|   Analog Devices INC.
|   IBIS Model of BF527/BF525/BF523
|   Embedded processor
|   208 Pin 17x17 CSP_BGA
[IBIS ver]   3.2
[File name]   bf527_1p8_17x17.ibs
[File Rev]   1.0
[Date]   02/23/2009
[Source]   From running Hspice on 90nm spice models.
[Notes]
|   Model data reflects 1.8v I/O Operation
|   No models exist for the following pins (Using type NC as
|   a placeholder):
|   XTAL, CLKIN, RTXI, RTXO, USB_ID, USB_DP, USB_XTALOUT,
|   USB_VBUS, USB_DM, VRSEL, USB_XTALIN, VROUT/EXT_WAKE1,
|   SS/PG, USB_RSET, USB_VREF
[Disclaimer]
|   This IBIS model is provided "AS IS, WHERE IS", AND WITH NO WARRANTY OF
|   ANY KIND EITHER EXPRESSED OR IMPLIED, INCLUDING BUT NOT LIMITED TO ANY
|   IMPLIED WARRANTIES OF MERCHANTABILITY AND FITNESS FOR A PARTICULAR
|   PURPOSE.  IN NO EVENT WILL ADI BE LIABLE FOR SPECIAL, COLLATERAL,
|   INCIDENTAL, OR CONSEQUENTIAL DAMAGES IN CONNECTION WITH OR ARISING OUT
|   OF THE USE OF THIS IBIS MODEL, AND IN NO EVENT SHALL ADI'S TOTAL
|   LIABILITY EXCEED $1,000, REGARDLESS OF THE BASIS FOR CLAIM.  ADI
|   RESERVES THE right to make changes to the products and IBIS models
|   without prior notice.
[Copyright]   This model is exclusive property of Analog Devices Inc
|   and is not to be resold or redistributed without the written
|   permission of Analog Devices.
|   Copyright (C)2008 Analog Devices, All Rights Reserved
[Component]   BF527/BF525/BF523
[Manufacturer] ANALOG DEVICES
[Package]
| variable   typ   min   max
R_pkg   217.00m   NA   NA
L_pkg   6.17nH   NA   NA
C_pkg   1.08pF   NA   NA
[Pin]   signal_name   model_name   R_pin   L_pin   C_pin
A1   GND   GND   NA   NA   NA
A2   PF9   prw0812swcdg_25   NA   NA   NA
A3   PF11   prw0408swcdg_25   NA   NA   NA
A4   SCL   piic400kv123   NA   NA   NA
A5   PF13   prw0812swcdg_25   NA   NA   NA
A6   PF15   prw0408swcdg_25   NA   NA   NA
A7   PH0   prw0408swcdg_25   NA   NA   NA
A8   PH2   prw0408swcdg_25   NA   NA   NA
A9   PH4   prw0408swcdg_25   NA   NA   NA
A10   XTAL   NC   NA   NA   NA
A11   CLKIN   NC   NA   NA   NA
A12   PH8   prw0408swcdg_25   NA   NA   NA
A13   PH10   prw0408swcdg_25   NA   NA   NA
A14   RTXI   NC   NA   NA   NA
A15   RTXO   NC   NA   NA   NA
A16   VDDRTC   POWER   NA   NA   NA
A17   GND   GND   NA   NA   NA
A18   USB_XTALOUT   NC   NA   NA   NA
A19   USB_XTALIN   NC   NA   NA   NA
A20   GND   GND   NA   NA   NA
B1   PF7   prw0408swcdg_25   NA   NA   NA
B2   PF8   prw0408swcdg_25   NA   NA   NA
B3   PF10   prw0408swcdg_25   NA   NA   NA
B4   SDA   piic400kv123   NA   NA   NA
B5   PF12   prw0408swcdg_25   NA   NA   NA
B6   PF14   prw0408swcdg_25   NA   NA   NA
B7   PH1   prw0408swcdg_25   NA   NA   NA
B8   PH3   prw0408swcdg_25   NA   NA   NA
B9   PH5   prw0408swcdg_25   NA   NA   NA
B10   PH6   prw0408swcdg_25   NA   NA   NA
B11   PH7   prw0408swcdg_25   NA   NA   NA
B12   PH9   prw0408swcdg_25   NA   NA   NA
B13   PH11   prw0408swcdg_25   NA   NA   NA
B14   PH12   prw0408swcdg_25   NA   NA   NA
B15   PH13   prw0408swcdg_25   NA   NA   NA
B16   PH14   prw0408swcdg_25   NA   NA   NA
B17   PH15   prw0408swcdg_25   NA   NA   NA
B18   RESET   prw0408swcdg_3v_25   NA   NA   NA
B19   NMI   prw0408swcdg_25   NA   NA   NA
B20   GND   GND   NA   NA   NA
C1   PF5   prw0812swcdg_25   NA   NA   NA
C2   PF6   prw0408swcdg_25   NA   NA   NA
C19   CLKBUF   prw0408swcdg_3v_25   NA   NA   NA
C20   USB_ID   NC   NA   NA   NA
D1   PF3   prw0408swcdg_25   NA   NA   NA
D2   PF4   prw0408swcdg_25   NA   NA   NA
D19   VDDUSB   POWER   NA   NA   NA
D20   USB_RSET   NC   NA   NA   NA
E1   PF1   prw0408swcdg_25   NA   NA   NA
E2   PF2   prw0812swcdg_25   NA   NA   NA
E19   USB_VBUS   NC   NA   NA   NA
E20   USB_DP   NC   NA   NA   NA
F1   PF0   prw0408swcdg_25   NA   NA   NA
F2   PPIFS1/TMR0   prw0408swcdg_25   NA   NA   NA
F19   VRSEL   NC   NA   NA   NA
F20   USB_DM   NC   NA   NA   NA
G1   PG15   prw0408swcdg_3v_25   NA   NA   NA
G2   PPICLK/TMRCLK  prw0408swcdg_25   NA   NA   NA
G7   VDDEXT   POWER   NA   NA   NA
G8   VDDEXT   POWER   NA   NA   NA
G9   VDDEXT   POWER   NA   NA   NA
G10   VDDEXT   POWER   NA   NA   NA
G11   VDDEXT   POWER   NA   NA   NA
G12   VDDINT   POWER   NA   NA   NA
G13   VDDINT   POWER   NA   NA   NA
G14   VDDINT   POWER   NA   NA   NA
G19   SS/PG   NC   NA   NA   NA
G20   VDDUSB   POWER   NA   NA   NA
H1   PG13   prw0408swcdg_25   NA   NA   NA
H2   PG14   prw0812swcdg_25   NA   NA   NA
H7   VDDEXT   POWER   NA   NA   NA
H8   VDDEXT   POWER   NA   NA   NA
H9   GND   GND   NA   NA   NA
H10   GND   GND   NA   NA   NA
H11   GND   GND   NA   NA   NA
H12   GND   GND   NA   NA   NA
H13   GND   GND   NA   NA   NA
H14   VDDINT   POWER   NA   NA   NA
H19   USB_VREF   NC   NA   NA   NA
H20   VROUT/EXT_WAKE1 NC   NA   NA   NA
J1   PG11   prw0408swcdg_25   NA   NA   NA
J2   PG12   prw0408swcdg_25   NA   NA   NA
J7   VDDEXT   POWER   NA   NA   NA
J8   VDDEXT   POWER   NA   NA   NA
J9   GND   GND   NA   NA   NA
J10   GND   GND   NA   NA   NA
J11   GND   GND   NA   NA   NA
J12   GND   GND   NA   NA   NA
J13   GND   GND   NA   NA   NA
J14   VDDINT   POWER   NA   NA   NA
J19   AMS0   prw1216cdg_25   NA   NA   NA
J20   EXT_WAKE2   prw0408swcdg_3v_25   NA   NA   NA
K1   PG9   prw0812swcdg_25   NA   NA   NA
K2   PG10   prw0812swcdg_25   NA   NA   NA
K7   VDDEXT   POWER   NA   NA   NA
K8   VDDEXT   POWER   NA   NA   NA
K9   GND   GND   NA   NA   NA
K10   GND   GND   NA   NA   NA
K11   GND   GND   NA   NA   NA
K12   GND   GND   NA   NA   NA
K13   GND   GND   NA   NA   NA
K14   VDDINT   POWER   NA   NA   NA
K19   AMS1   prw1216cdg_25   NA   NA   NA
K20   CLKOUT   prw1624cdg_25   NA   NA   NA
L1   PG7   prw0408swcdg_25   NA   NA   NA
L2   PG8   prw0408swcdg_25   NA   NA   NA
L7   VDDEXT   POWER   NA   NA   NA
L8   VDDMEM   POWER   NA   NA   NA
L9   GND   GND   NA   NA   NA
L10   GND   GND   NA   NA   NA
L11   GND   GND   NA   NA   NA
L12   GND   GND   NA   NA   NA
L13   GND   GND   NA   NA   NA
L14   VDDINT   POWER   NA   NA   NA
L19   VPPOTP   POWER   NA   NA   NA
L20   AMS3   prw1216cdg_25   NA   NA   NA
M1   PG5   prw0408swcdg_25   NA   NA   NA
M2   PG6   prw0408swcdg_25   NA   NA   NA
M7   VDDMEM   POWER   NA   NA   NA
M8   VDDMEM   POWER   NA   NA   NA
M9   GND   GND   NA   NA   NA
M10   GND   GND   NA   NA   NA
M11   GND   GND   NA   NA   NA
M12   GND   GND   NA   NA   NA
M13   GND   GND   NA   NA   NA
M14   VDDINT   POWER   NA   NA   NA
M19   AMS2   prw1216cdg_25   NA   NA   NA
M20   ARE   prw1216cdg_25   NA   NA   NA
N1   PG3   prw0408swcdg_25   NA   NA   NA
N2   PG4   prw0408swcdg_25   NA   NA   NA
N7   VDDMEM   POWER   NA   NA   NA
N8   VDDMEM   POWER   NA   NA   NA
N9   GND   GND   NA   NA   NA
N10   GND   GND   NA   NA   NA
N11   GND   GND   NA   NA   NA
N12   GND   GND   NA   NA   NA
N13   GND   GND   NA   NA   NA
N14   VDDINT   POWER   NA   NA   NA
N19   AWE   prw1216cdg_25   NA   NA   NA
N20   AOE   prw1216cdg_25   NA   NA   NA
P1   PG1   prw0408swcdg_25   NA   NA   NA
P2   PG2   prw0812swcdg_25   NA   NA   NA
P7   VDDMEM   POWER   NA   NA   NA
P8   VDDMEM   POWER   NA   NA   NA
P9   VDDMEM   POWER   NA   NA   NA
P10   VDDMEM   POWER   NA   NA   NA
P11   VDDMEM   POWER   NA   NA   NA
P12   VDDINT   POWER   NA   NA   NA
P13   VDDINT   POWER   NA   NA   NA
P14   VDDINT   POWER   NA   NA   NA
P19   ARDY   prw1216cdg_25   NA   NA   NA
P20   SCKE   prw1216cdg_25   NA   NA   NA
R1   TDI   prwd0408swcdg_25   NA   NA   NA
R2   PG0   prw0408swcdg_25   NA   NA   NA
R19   SMS   prw1216cdg_25   NA   NA   NA
R20   VDDOTP   POWER   NA   NA   NA
T1   TDO   prw0408swcdg_25   NA   NA   NA
T2   EMU   prw0408swcdg_25   NA   NA   NA
T19   SRAS   prw1216cdg_25   NA   NA   NA
T20   SWE   prw1216cdg_25   NA   NA   NA
U1   TRST   prwd0408swcdg_25   NA   NA   NA
U2   TMS   prwd0408swcdg_25   NA   NA   NA
U19   SA10   prw1216cdg_25   NA   NA   NA
U20   SCAS   prw1216cdg_25   NA   NA   NA
V1   DATA15   prw1216hcdg_25   NA   NA   NA
V2   TCK   prwd0408swcdg_25   NA   NA   NA
V19   ABE0/SDQM0  prw1216cdg_25   NA   NA   NA
V20   ABE1/SDQM1  prw1216cdg_25   NA   NA   NA
W1   DATA14   prw1216hcdg_25   NA   NA   NA
W2   DATA13   prw1216hcdg_25   NA   NA   NA
W3   DATA11   prw1216hcdg_25   NA   NA   NA
W4   DATA9   prw1216hcdg_25   NA   NA   NA
W5   DATA7   prw1216hcdg_25   NA   NA   NA
W6   DATA5   prw1216hcdg_25   NA   NA   NA
W7   DATA3   prw1216hcdg_25   NA   NA   NA
W8   DATA1   prw1216hcdg_25   NA   NA   NA
W9   BMODE3   prw0408swcdg_25   NA   NA   NA
W10   BMODE1   prw0408swcdg_25   NA   NA   NA
W11   ADDR18   prw1216cdg_25   NA   NA   NA
W12   ADDR16   prw1216cdg_25   NA   NA   NA
W13   ADDR14   prw1216cdg_25   NA   NA   NA
W14   ADDR12   prw1216cdg_25   NA   NA   NA
W15   ADDR10   prw1216cdg_25   NA   NA   NA
W16   ADDR8   prw1216cdg_25   NA   NA   NA
W17   ADDR6   prw1216cdg_25   NA   NA   NA
W18   ADDR4   prw1216cdg_25   NA   NA   NA
W19   ADDR2   prw1216cdg_25   NA   NA   NA
W20   ADDR1   prw1216cdg_25   NA   NA   NA
Y1   GND   GND   NA   NA   NA
Y2   DATA12   prw1216hcdg_25   NA   NA   NA
Y3   DATA10   prw1216hcdg_25   NA   NA   NA
Y4   DATA8   prw1216hcdg_25   NA   NA   NA
Y5   DATA6   prw1216hcdg_25   NA   NA   NA
Y6   DATA4   prw1216hcdg_25   NA   NA   NA
Y7   DATA2   prw1216hcdg_25   NA   NA   NA
Y8   DATA0   prw1216hcdg_25   NA   NA   NA
Y9   BMODE2   prw0408swcdg_25   NA   NA   NA
Y10   BMODE0   prw0408swcdg_25   NA   NA   NA
Y11   ADDR19   prw1216cdg_25   NA   NA   NA
Y12   ADDR17   prw1216cdg_25   NA   NA   NA
Y13   ADDR15   prw1216cdg_25   NA   NA   NA
Y14   ADDR13   prw1216cdg_25   NA   NA   NA
Y15   ADDR11   prw1216cdg_25   NA   NA   NA
Y16   ADDR9   prw1216cdg_25   NA   NA   NA
Y17   ADDR7   prw1216cdg_25   NA   NA   NA
Y18   ADDR5   prw1216cdg_25   NA   NA   NA
Y19   ADDR3   prw1216cdg_25   NA   NA   NA
Y20   GND   GND   NA   NA   NA
[Model Selector]   prw0408swcdg_25
COUT_8 8mA buffer
[Model Selector]   prwd0408swcdg_25
EOUT_8 8mA buffer
[Model Selector]   prw0408swcdg_3v_25
FOUT_8 8mA buffer
[Model Selector]   prw0812swcdg_25
IOUT_12 12mA buffer
[Model Selector]   prw1216cdg_25
MOUT_16 16mA buffer
[Model Selector]   prw1216hcdg_25
NOUT_16 16mA buffer
[Model Selector]   prw1624cdg_25
QOUT_24 24mA buffer
[Model Selector]   piic400kv123
twi_s5 Vbus 1.8V
twi_s6 Vbus 2.5V
twi_s7 Vbus 3.3V
| Models and submodels in the file (10): twi_s5 (I/O_open_drain), twi_s6 (I/O_open_drain), twi_s7 (I/O_open_drain), COUT_8 (I/O), FOUT_8 (I/O), IOUT_12 (I/O), MOUT_16 (I/O), NOUT_16 (I/O), EOUT_8 (I/O), QOUT_24 (I/O)
